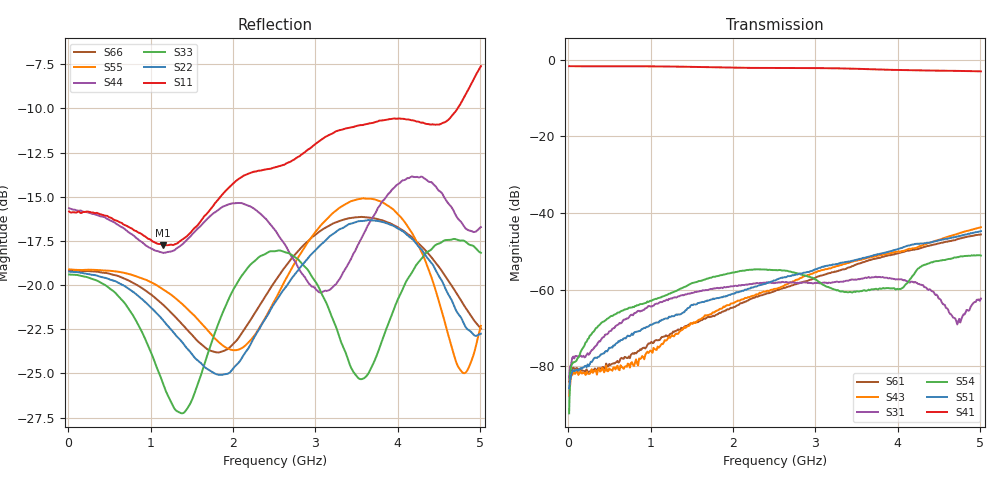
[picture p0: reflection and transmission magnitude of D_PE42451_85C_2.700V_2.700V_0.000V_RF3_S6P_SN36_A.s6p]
! Device ID: PE42451
! Serial: 36
! Insertion: A
! Temp: 85C
! VDD: 2.700
! Control_Hi: 100.000
! Control_Lo: 0.000
! Logic State: RF3
! Port 1: RFC
! Port 2: RF1
! Port 3: RF2
! Port 4: RF3
! Port 5: RF4
! Port 6: RF5
! V1 = 2.70
! V2 = 2.70
! V3 = 0.00
! V4 = 0.00
! IDD: 1.127000e-05
#  Hz  S  RI  R  50
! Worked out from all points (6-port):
!   401 points, 10 MHz to 5.01 GHz, reference 50 ohm
!   strongest paths, dB at 10 MHz, 1.26 GHz, 2.51 GHz, 3.76 GHz, 5.01 GHz:
!     S41: -1.7, -1.8, -2.1, -2.5, -3.0
!     S51: -85.7, -66.9, -57.6, -50.7, -44.7
!     S54: -92.2, -60.8, -54.9, -59.9, -51.1
!     S31: -82.9, -62.3, -58.2, -56.7, -62.3
!     S43: -87.6, -71.8, -59.8, -51.1, -43.7
!     S61: -84.0, -71.4, -60.4, -51.7, -45.6
!   lowest |S11| = -17.8 dB at 1.147 GHz (marker M1), VSWR 1.30, Z = 58.1 - j11.5 ohm
!   |S11| at or under -10 dB: start of sweep to 4.728 GHz
